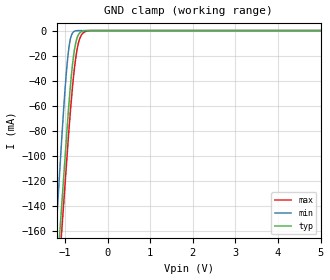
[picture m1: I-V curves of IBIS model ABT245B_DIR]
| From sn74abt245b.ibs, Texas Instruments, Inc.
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[Model]   ABT245B_DIR
Model_type  Input
Vinl=0.8
Vinh=2.0
| variable   typ   min   max
C_comp   2.94pF   2.29pF   4.54pF
[Temperature Range]   40   -40   100
| Ambient temperature   25   -40   85
[Voltage range]   5   4.5   5.5
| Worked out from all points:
|   GND clamp passes 1 mA (typ) near -0.62 V on its own axis
[GND Clamp]
| ABT245B_DIR
|   Voltage   I(typ)   I(min)   I(max)
-5V       -2.044A    -2.268A    -2.043A
-1.215V   -205.9mA   -162.5mA   -226.1mA
-1.125V   -162.3mA   -112.7mA   -183mA
-1.075V   -138.1mA   -85mA      -159mA
-1V       -101.8mA   -47.03mA   -123.1mA
-925mV    -65.85mA   -17.87mA   -87.12mA
-850mV    -35.5mA    -3.716mA   -54.7mA
-775mV    -14.49mA   -457.1uA   -28.95mA
-725mV    -6.598mA   -67.08uA   -16.6mA
-650mV    -1.663mA   -1.978uA   -5.929mA
-450mV    -7.799uA   -255.4pA   -194.7uA
5V        31.82pA    20.18pA    969.5pA
